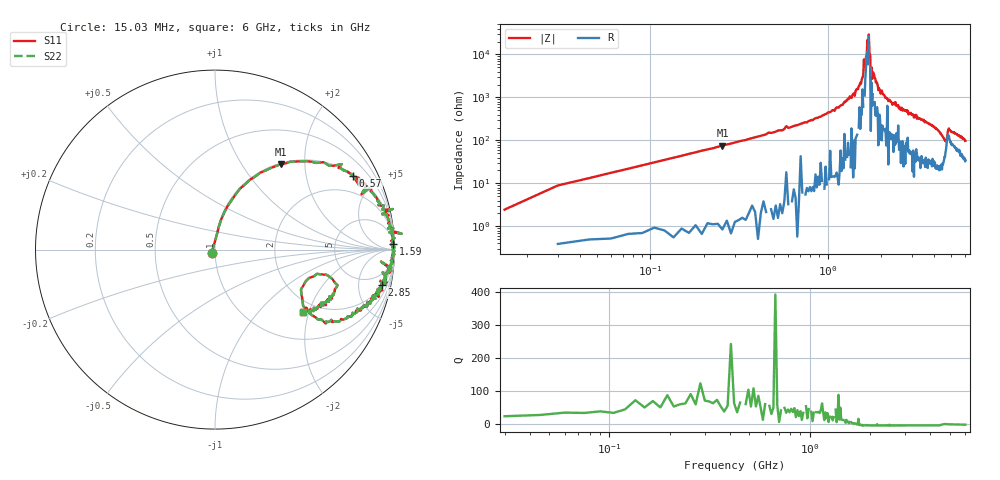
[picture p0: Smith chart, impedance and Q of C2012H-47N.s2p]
!	Network	Analyzer	HP8753E.07.74:	Oct	30	2002	Serial	No.	JP38451487
!	Hewlett-Packard
!	28	Aug	2009	10:16:09
!	Frequency	S11	S21	S12	S22
#	HZ	S	RI	R	50
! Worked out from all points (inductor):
!   400 points, 15.03 MHz to 6 GHz, reference 50 ohm
!   read as one part in series: L = 46.8 nH near 45.03 MHz
!   highest Q = 67.8 at 255 MHz (marker M1), where L = 47.6 nH
!   self-resonance near 1.65 GHz
!   S11 on the Smith chart (normalised r, x): 15.03 MHz: 0.96, -0.03; 570 MHz: 1.08, +3.69; 1.59 GHz: 14, +63; 2.85 GHz: 2.24, -8.99; 6 GHz: 1.68, -1.84
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1.502992e7  -0.0181 -0.0163  1.02 0.0163  1.02 0.0163  -0.0181 -0.0163
3.002985e7  0.0115 0.0881  0.988 -0.0881  0.988 -0.0881  0.0115 0.0881
7.502962e7  0.0517 0.207  0.948 -0.207  0.948 -0.207  0.0517 0.207
2.550287e8  0.369 0.477  0.631 -0.477  0.631 -0.477  0.369 0.477
5.700272e8  0.768 0.412  0.232 -0.412  0.232 -0.412  0.768 0.412
1.020025e9  0.948 0.209  0.0522 -0.209  0.0522 -0.209  0.948 0.209
1.590022e9  0.993 0.03  0.00665 -0.03  0.00665 -0.03  0.993 0.03
1.605022e9  1 0.0127  -0.00286 -0.0127  -0.00286 -0.0127  1 0.0127
1.635022e9  0.987 0.0166  0.0131 -0.0166  0.0131 -0.0166  0.987 0.0166
1.680022e9  0.998 0.00391  0.00235 -0.00391  0.00235 -0.00391  0.998 0.00391
1.695022e9  0.993 0.0083  0.0072 -0.0083  0.0072 -0.0083  0.993 0.0083
1.710021e9  0.997 -0.00153  0.00305 0.00153  0.00305 0.00153  0.997 -0.00153
1.740021e9  0.995 -0.00873  0.00507 0.00873  0.00507 0.00873  0.995 -0.00873
1.755021e9  0.996 0.0391  0.00412 -0.0391  0.00412 -0.0391  0.996 0.0391
1.770021e9  0.991 -0.0174  0.00885 0.0174  0.00885 0.0174  0.991 -0.0174
1.785021e9  0.99 -0.0353  0.00989 0.0353  0.00989 0.0353  0.99 -0.0353
2.01002e9  0.983 -0.0706  0.0172 0.0706  0.0172 0.0706  0.983 -0.0706
2.850016e9  0.929 -0.197  0.0711 0.197  0.0711 0.197  0.929 -0.197
3.015015e9  0.933 -0.228  0.0673 0.228  0.0673 0.228  0.933 -0.228
4.00501e9  0.778 -0.357  0.222 0.357  0.222 0.357  0.778 -0.357
5.010005e9  0.651 -0.26  0.349 0.26  0.349 0.26  0.651 -0.26
6e9  0.493 -0.348  0.507 0.348  0.507 0.348  0.493 -0.348
